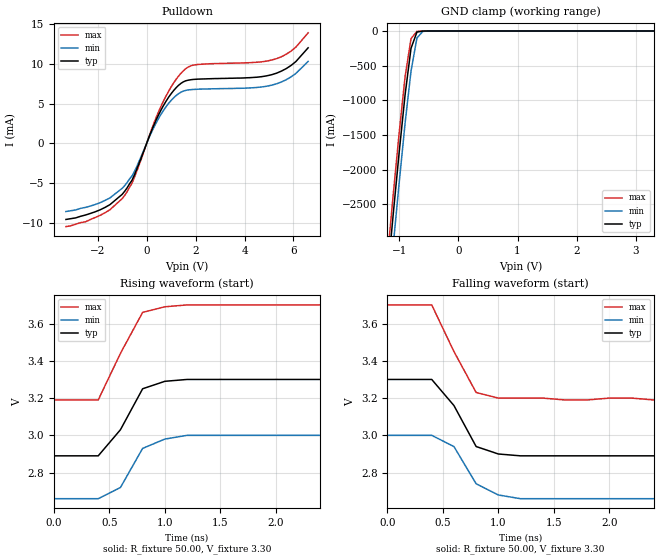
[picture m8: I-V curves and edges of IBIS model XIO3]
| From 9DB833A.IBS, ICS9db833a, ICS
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|   Model XIO3
[Model]   XIO3
Model_type   I/O_open_drain
Polarity   Inverting
Enable   Active-High
Vinl =   0.80V
Vinh =   2.00V
Vmeas =   1.50V
Cref =  30.00pF
Rref =  2700.000
Vref =   1.50V
C_comp   3.40pF   2.85pF   3.95pF
[Temperature Range]   27.00   70.00   0.00
[Voltage Range]   3.30V   3.00V   3.70V
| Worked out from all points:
|   slope of the pulldown table from 0 to 0.495 V, typ, clamps not added: 136 ohm
|   GND clamp passes 1 mA (typ) near -0.60 V on its own axis
|   rising waveform, R_fixture 50.00, V_fixture 3.30: 20-80 % time 254ps typ, 200ps min, 262ps max; typ from 2.89 V to 3.3 V
|   falling waveform, R_fixture 50.00, V_fixture 3.30: 20-80 % time 254ps typ, 232ps min, 262ps max; typ from 3.3 V to 2.89 V
[Pulldown]
| voltage   I(typ)   I(min)   I(max)
-3.3V     -9.6mA     -8.6mA     -10.5mA
-1.9V     -8.38mA    -7.48mA    -9.08mA
-900mV    -6.05mA    -5.34mA    -6.57mA
-600mV    -4.66mA    -4.12mA    -5.04mA
300mV     2.34mA     2.05mA     2.57mA
700mV     4.84mA     4.21mA     5.42mA
1.2V      7mA        6.02mA     8.06mA
1.6V      7.89mA     6.68mA     9.42mA
2.1V      8.1mA      6.83mA     9.95mA
5.1V      8.65mA     7.33mA     10.5mA
5.9V      9.82mA     8.38mA     11.63mA
6.6V      12.05mA    10.33mA    13.94mA
[GND_clamp]
| voltage   I(typ)   I(min)   I(max)
-3.3V     -24.06A    -24.47A    -23.81A
-1.2V     -3.56A     -4.01A     -3.28A
-1.1V     -2.64A     -3.09A     -2.36A
-1V       -1.75A     -2.19A     -1.47A
-900mV    -920mA     -1.33A     -660mA
-800mV    -250mA     -580mA     -110mA
-700mV    -15.36mA   -100mA     -4.21mA
-600mV    -910uA     -5.53mA    -470uA
-500mV    -90.77uA   -340uA     -47.47uA
3.3V      130pA      330pA      120pA
[Ramp]
| variable   typ   min   max
dV/dt_r   0.25/0.19n   0.21/0.17n   0.30/0.17n
dV/dt_f   0.25/0.19n   0.21/0.19n   0.30/0.17n
R_load = 50.00
[Rising Waveform]
R_fixture = 50.00
V_fixture = 3.30
V_fixture_min = 3.00
V_fixture_max = 3.70
| time   V(typ)   V(min)   V(max)
0s        2.89V      2.66V      3.19V
400ps     2.89V      2.66V      3.19V
600ps     3.03V      2.72V      3.44V
800ps     3.25V      2.93V      3.66V
1ns       3.29V      2.98V      3.69V
1.2ns     3.3V       3V         3.7V
10ns      3.3V       3V         3.7V
[Falling Waveform]
R_fixture = 50.00
V_fixture = 3.30
V_fixture_min = 3.00
V_fixture_max = 3.70
| time   V(typ)   V(min)   V(max)
0s        3.3V       3V         3.7V
400ps     3.3V       3V         3.7V
600ps     3.16V      2.94V      3.45V
800ps     2.94V      2.74V      3.23V
1ns       2.9V       2.68V      3.2V
1.2ns     2.89V      2.66V      3.2V
1.6ns     2.89V      2.66V      3.19V
2ns       2.89V      2.66V      3.2V
2.4ns     2.89V      2.66V      3.19V
10ns      2.89V      2.66V      3.19V
